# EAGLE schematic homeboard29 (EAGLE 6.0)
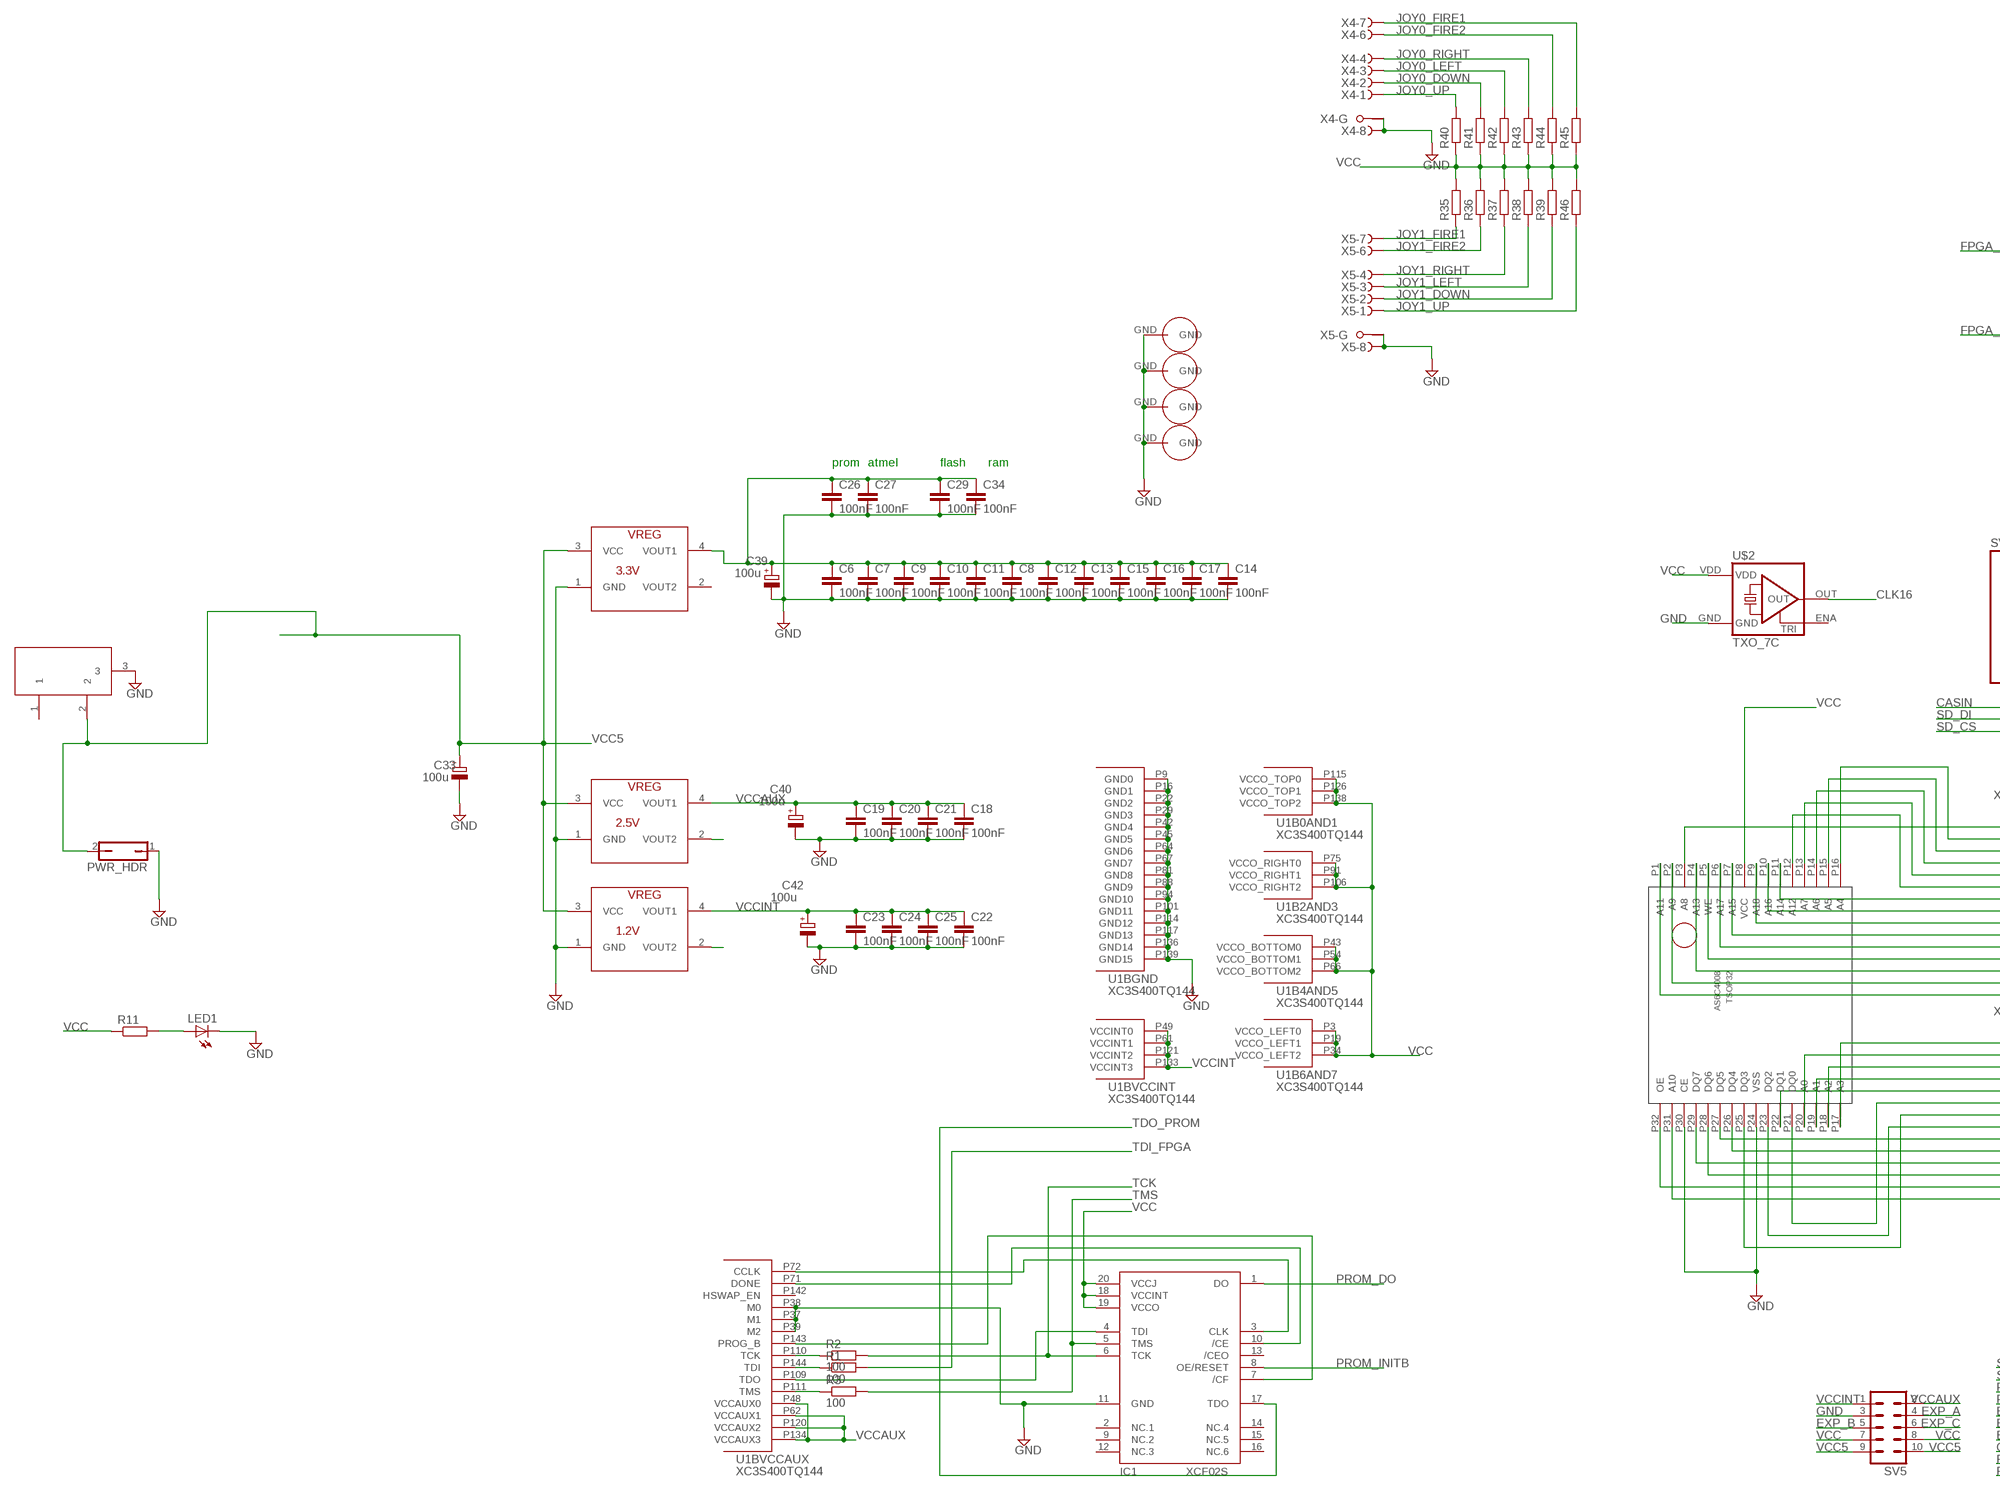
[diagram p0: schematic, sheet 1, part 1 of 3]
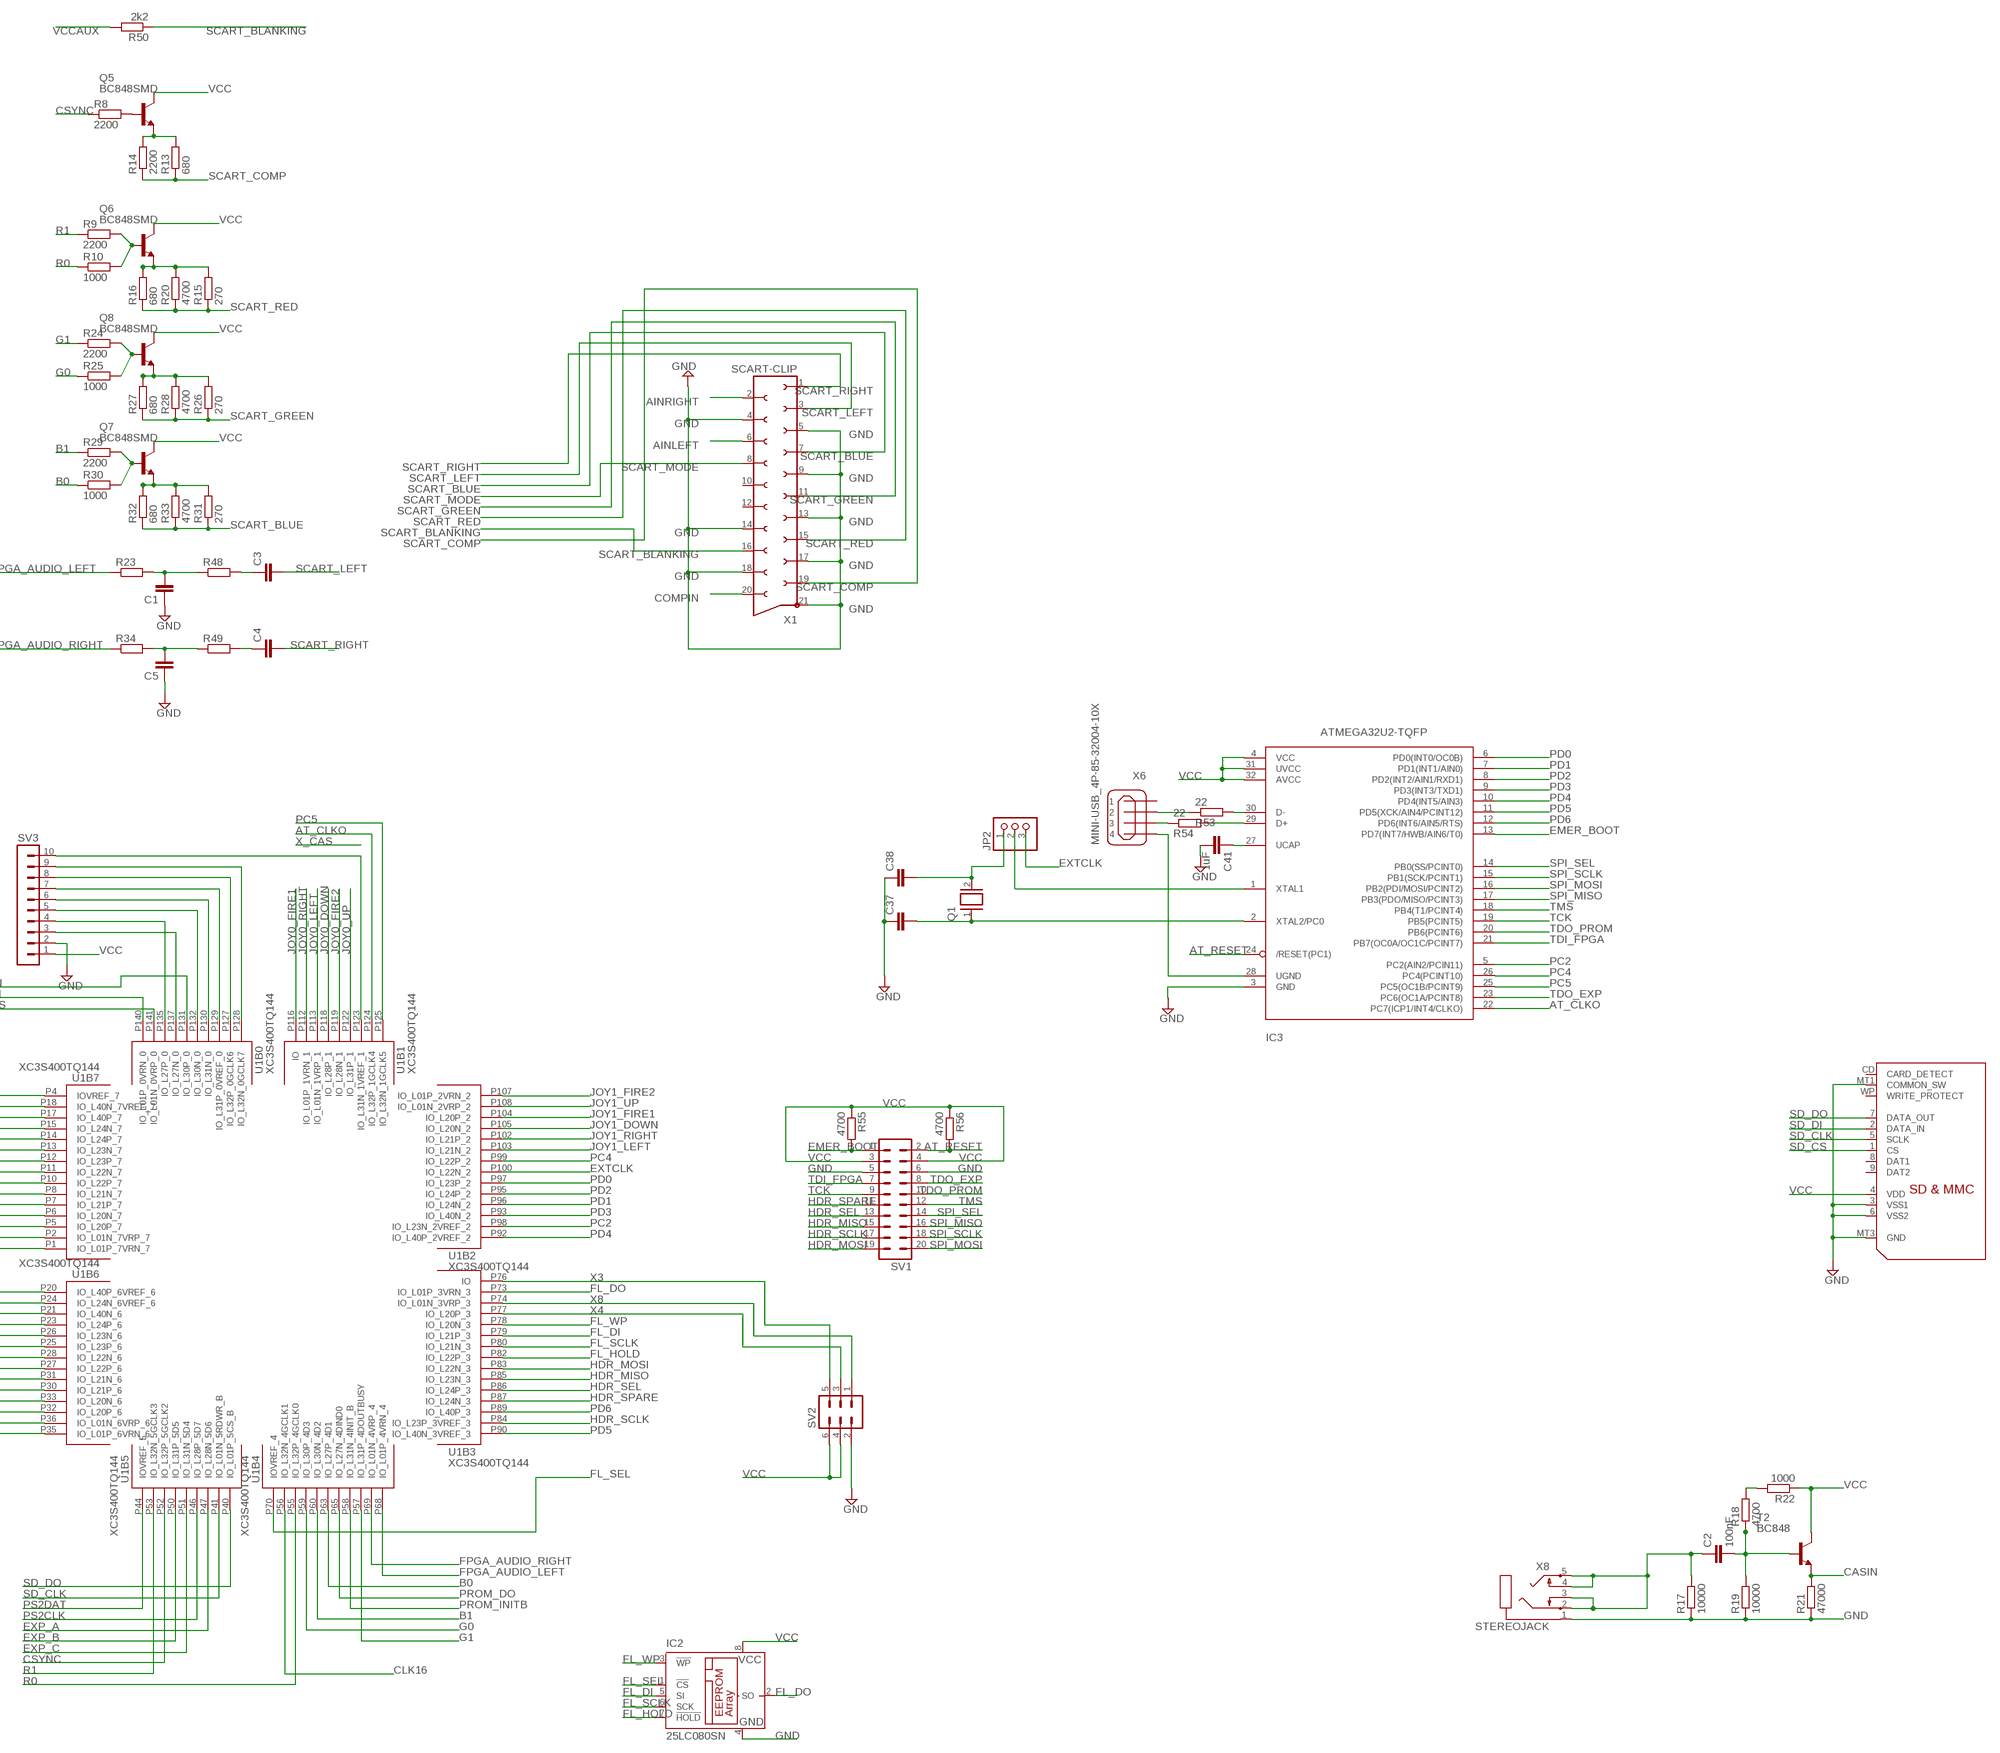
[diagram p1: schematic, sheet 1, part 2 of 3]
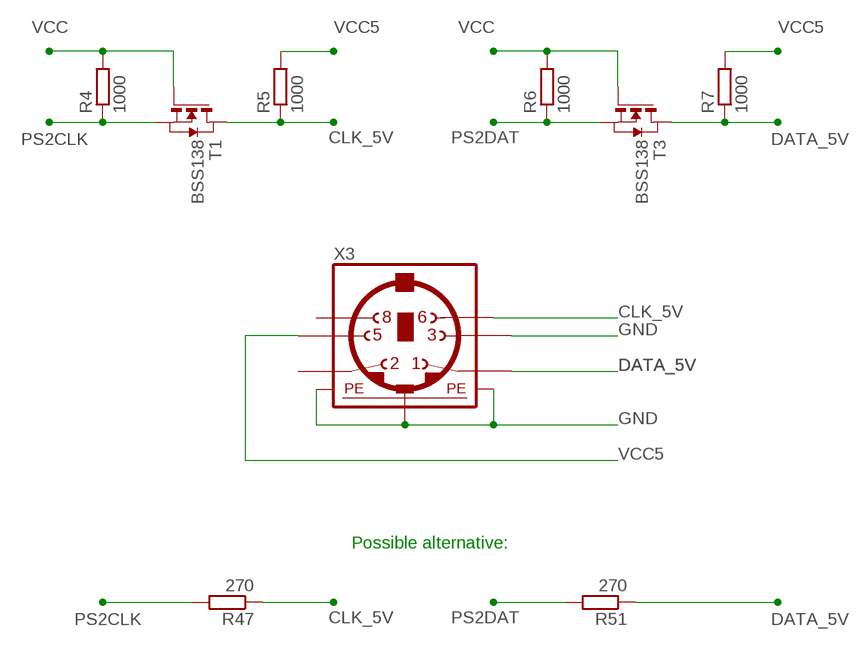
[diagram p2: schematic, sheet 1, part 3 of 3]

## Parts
C1  C-EUC0603  [C0603]
C2  100nF  C-EUC0603  [C0603]
C3  C-EUC0603  [C0603]
C4  C-EUC0603  [C0603]
C5  C-EUC0603  [C0603]
C6  100nF  C-EUC0603  [C0603]
C7  100nF  C-EUC0603  [C0603]
C8  100nF  C-EUC0603  [C0603]
C9  100nF  C-EUC0603  [C0603]
C10  100nF  C-EUC0603  [C0603]
C11  100nF  C-EUC0603  [C0603]
C12  100nF  C-EUC0603  [C0603]
C13  100nF  C-EUC0603  [C0603]
C14  100nF  C-EUC0603  [C0603]
C15  100nF  C-EUC0603  [C0603]
C16  100nF  C-EUC0603  [C0603]
C17  100nF  C-EUC0603  [C0603]
C18  100nF  C-EUC0603  [C0603]
C19  100nF  C-EUC0603  [C0603]
C20  100nF  C-EUC0603  [C0603]
C21  100nF  C-EUC0603  [C0603]
C22  100nF  C-EUC0603  [C0603]
C23  100nF  C-EUC0603  [C0603]
C24  100nF  C-EUC0603  [C0603]
C25  100nF  C-EUC0603  [C0603]
C26  100nF  C-EUC0603  [C0603]
C27  100nF  C-EUC0603  [C0603]
C29  100nF  C-EUC0603  [C0603]
C33  100u  CPOL-EUD  [PANASONIC_D]
C34  100nF  C-EUC0603  [C0603]
C37  C-EUC0805  [C0805]
C38  C-EUC0805  [C0805]
C39  100u  CPOL-EUD  [PANASONIC_D]
C40  100u  CPOL-EUD  [PANASONIC_D]
C41  1uF  C-EUC0805  [C0805]
C42  100u  CPOL-EUD  [PANASONIC_D]
IC1  XCF02S  [VO20]
IC2  25LC080SN  [SO-08]
IC3  ATMEGA32U2-TQFP  [TQFP32-08]
JP2  PINHD-1X3  [1X03]
LED1  LEDCHIPLED_0805  [CHIPLED_0805]
PWR_HDR  JP1Q  [JP1]
Q1  XTAL/S  [QS]
Q5  BC848SMD  [SOT23]
Q6  BC848SMD  [SOT23]
Q7  BC848SMD  [SOT23]
Q8  BC848SMD  [SOT23]
R1  100  R-EU_R0805  [R0805]
R2  100  R-EU_R0805  [R0805]
R3  100  R-EU_R0805  [R0805]
R4  1000  R-EU_R0805  [R0805]
R5  1000  R-EU_R0805  [R0805]
R6  1000  R-EU_R0805  [R0805]
R7  1000  R-EU_R0805  [R0805]
R8  2200  R-EU_R0805  [R0805]
R9  2200  R-EU_R0805  [R0805]
R10  1000  R-EU_R0805  [R0805]
R11  R-EU_M0805  [M0805]
R13  680  R-EU_R0805  [R0805]
R14  2200  R-EU_R0805  [R0805]
R15  270  R-EU_R0805  [R0805]
R16  680  R-EU_R0805  [R0805]
R17  10000  R-EU_R0805  [R0805]
R18  4700  R-EU_R0805  [R0805]
R19  10000  R-EU_R0805  [R0805]
R20  4700  R-EU_R0805  [R0805]
R21  47000  R-EU_R0805  [R0805]
R22  1000  R-EU_R0805  [R0805]
R23  R-EU_M0805  [M0805]
R24  2200  R-EU_R0805  [R0805]
R25  1000  R-EU_R0805  [R0805]
R26  270  R-EU_R0805  [R0805]
R27  680  R-EU_R0805  [R0805]
R28  4700  R-EU_R0805  [R0805]
R29  2200  R-EU_R0805  [R0805]
R30  1000  R-EU_R0805  [R0805]
R31  270  R-EU_R0805  [R0805]
R32  680  R-EU_R0805  [R0805]
R33  4700  R-EU_R0805  [R0805]
R34  R-EU_M0805  [M0805]
R35  R-EU_M0805  [M0805]
R36  R-EU_M0805  [M0805]
R37  R-EU_M0805  [M0805]
R38  R-EU_M0805  [M0805]
R39  R-EU_M0805  [M0805]
R40  R-EU_M0805  [M0805]
R41  R-EU_M0805  [M0805]
R42  R-EU_M0805  [M0805]
R43  R-EU_M0805  [M0805]
R44  R-EU_M0805  [M0805]
R45  R-EU_M0805  [M0805]
R46  R-EU_M0805  [M0805]
R47  270  R-EU_R0805  [R0805]
R48  R-EU_M0805  [M0805]
R49  R-EU_M0805  [M0805]
R50  2k2  R-EU_M0805  [M0805]
R51  270  R-EU_R0805  [R0805]
R53  22  R-EU_R0805  [R0805]
R54  22  R-EU_R0805  [R0805]
R55  4700  R-EU_R0805  [R0805]
R56  4700  R-EU_R0805  [R0805]
REG1.2  1.2V  NX1117  [SOT223]
REG2.5  2.5V  NX1117  [SOT223]
REG3.3  3.3V  NX1117  [SOT223]
SV1  MA10-2  [MA10-2]
SV2  MA03-2  [MA03-2]
SV3  MA10-1  [MA10-1]
SV5  MA05-2  [MA05-2]
T1  BSS138  NMOSSOT23  [SOT-23]
T2  BC848  [SOT23]
T3  BSS138  NMOSSOT23  [SOT-23]
U1  XC3S400TQ144  [TQ144]
U$1  GNDHOLE  [GNDHOLE]
U$2  TXO_7C  [OSC_7C]
U$3  SDMMCNOHOLE  [SDCARD-NOHOLE]
U$6  AS6C4008  [TSOP32]
U$7  GNDHOLE  [GNDHOLE]
U$8  GNDHOLE  [GNDHOLE]
U$9  GNDHOLE  [GNDHOLE]
X1  SCART-CLIP  [SCART-CLIP]
X3  MINI_DIN_6  [M_DIN6]
X4  F09HPS  [F09HP]
X5  F09HPS  [F09HP]
X6  MINI-USB_4P-85-32004-10X  [85-32004-10X]
X7  DC21MMX  [DC-21MM]
X8  STEREOJACK  [20-0137]

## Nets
AINLEFT: X1.6
AINRIGHT: X1.2
AT_CLKO: IC3.22(PC7(ICP1/INT4/CLKO)) U1.P124(B1:IO_L32P_1GCLK4)
AT_RESET: IC3.24(/RESET(PC1)) R56.2 SV1.2
B0: R30.1 U1.P63(B4:IO_L27P_4D1)
B1: R29.1 U1.P60(B4:IO_L30N_4D2)
CASIN: R21.2 T2.2(E) U1.P131(B0:IO_L30P_0)
CLK16: U1.P56(B4:IO_L32N_4GCLK1) U$2.OUT
CLK_5V: R5.1 R47.1 T1.1(D) X3.6
COMPIN: X1.20
CSYNC: R8.1 U1.P52(B5:IO_L32P_5GCLK2)
DATA_5V: R7.1 R51.1 T3.1(D) X3.1
EMER_BOOT: IC3.13(PD7(INT7/HWB/AIN6/T0)) R55.2 SV1.1
EXP_A: SV5.4 U1.P47(B5:IO_L28N_5D6)
EXP_B: SV5.5 U1.P50(B5:IO_L31P_5D5)
EXP_C: SV5.6 U1.P51(B5:IO_L31N_5D4)
EXTCLK: JP2.3 U1.P100(B2:IO_L22N_2)
FL_DI: IC2.5(SI) U1.P79(B3:IO_L21P_3)
FL_DO: IC2.2(SO) U1.P73(B3:IO_L01P_3VRN_3)
FL_HOLD: IC2.7(!HOLD) U1.P82(B3:IO_L22P_3)
FL_SCLK: IC2.6(SCK) U1.P80(B3:IO_L21N_3)
FL_SEL: IC2.1(!CS) U1.P70(B4:IOVREF_4)
FL_WP: IC2.3(!WP) U1.P78(B3:IO_L20N_3)
FPGA_AUDIO_LEFT: R23.1 U1.P68(B4:IO_L01P_4VRN_4)
FPGA_AUDIO_RIGHT: R34.1 U1.P69(B4:IO_L01N_4VRP_4)
G0: R25.1 U1.P59(B4:IO_L30P_4D3)
G1: R24.1 U1.P57(B4:IO_L31P_4DOUTBUSY)
GND: C1.1 C5.1 C6.2 C7.2 C8.2 C9.2 C10.2 C11.2 C12.2 C13.2 C14.2 C15.2 C16.2 C17.2 C18.2 C19.2 C20.2 C21.2 C22.2 C23.2 C24.2 C25.2 C26.2 C27.2 C29.2 C33.- C34.2 C37.1 C38.1 C39.- C40.- C41.2 C42.- IC1.11(GND) IC2.4(GND) IC3.3(GND) LED1.C PWR_HDR.1 R17.1 R19.1 R21.1 REG1.2.1(GND) REG2.5.1(GND) REG3.3.1(GND) SV1.5 SV1.6 SV2.2 SV3.2 SV5.3 U1.P9(BGND:GND0) U1.P16(BGND:GND1) U1.P22(BGND:GND2) U1.P29(BGND:GND3) U1.P37(BVCCAUX:M1) U1.P38(BVCCAUX:M0) U1.P39(BVCCAUX:M2) U1.P42(BGND:GND4) U1.P45(BGND:GND5) U1.P64(BGND:GND6) U1.P67(BGND:GND7) U1.P81(BGND:GND8) U1.P88(BGND:GND9) U1.P94(BGND:GND10) U1.P101(BGND:GND11) U1.P114(BGND:GND12) U1.P117(BGND:GND13) U1.P136(BGND:GND14) U1.P139(BGND:GND15) U$1.GND U$2.GND U$3.3(VSS1) U$3.6(VSS2) U$3.MT1(COMMON_SW) U$3.MT3(GND) U$6.P24(VSS) U$6.P30(CE) U$7.GND U$8.GND U$9.GND X1.4 X1.5 X1.9 X1.13 X1.14 X1.17 X1.18 X1.21 X3.3 X3.SH1(PE1) X3.SH2(PE2) X3.SH3(PE3) X4.8(-8:F) X4.G1(-G:G1) X5.8(-8:F) X5.G1(-G:G1) X7.3 X8.1
HDR_MISO: SV1.15 U1.P85(B3:IO_L23N_3)
HDR_MOSI: SV1.19 U1.P83(B3:IO_L22N_3)
HDR_SCLK: SV1.17 U1.P84(B3:IO_L23P_3VREF_3)
HDR_SEL: SV1.13 U1.P86(B3:IO_L24P_3)
HDR_SPARE: SV1.11 U1.P87(B3:IO_L24N_3)
JOY0_DOWN: R41.2 U1.P118(B1:IO_L28P_1) X4.2(-2:F)
JOY0_FIRE1: R45.2 U1.P116(B1:IO) X4.7(-7:F)
JOY0_FIRE2: R44.2 U1.P119(B1:IO_L28N_1) X4.6(-6:F)
JOY0_LEFT: R42.2 U1.P113(B1:IO_L01N_1VRP_1) X4.3(-3:F)
JOY0_RIGHT: R43.2 U1.P112(B1:IO_L01P_1VRN_1) X4.4(-4:F)
JOY0_UP: R40.2 U1.P122(B1:IO_L31P_1) X4.1(-1:F)
JOY1_DOWN: R39.1 U1.P105(B2:IO_L20N_2) X5.2(-2:F)
JOY1_FIRE1: R35.1 U1.P104(B2:IO_L20P_2) X5.7(-7:F)
JOY1_FIRE2: R36.1 U1.P107(B2:IO_L01P_2VRN_2) X5.6(-6:F)
JOY1_LEFT: R38.1 U1.P103(B2:IO_L21N_2) X5.3(-3:F)
JOY1_RIGHT: R37.1 U1.P102(B2:IO_L21P_2) X5.4(-4:F)
JOY1_UP: R46.1 U1.P108(B2:IO_L01N_2VRP_2) X5.1(-1:F)
N$1: SV3.4 U1.P135(B0:IO_L27P_0)
N$2: SV3.5 U1.P132(B0:IO_L30N_0)
N$3: SV3.3 U1.P137(B0:IO_L27N_0)
N$4: SV3.6 U1.P130(B0:IO_L31N_0)
N$5: SV3.7 U1.P129(B0:IO_L31P_0VREF_0)
N$6: SV3.9 U1.P128(B0:IO_L32N_0GCLK7)
N$7: SV3.8 U1.P127(B0:IO_L32P_0GCLK6)
N$8: IC3.1(XTAL1) JP2.2
N$9: C41.1 IC3.27(UCAP)
N$10: LED1.A R11.2
N$12: C37.2 IC3.2(XTAL2/PC0) Q1.1
N$14: C38.2 JP2.1 Q1.2
N$16: SV3.10 U1.P123(B1:IO_L31N_1VREF_1)
N$35: IC1.3(CLK) U1.P72(BVCCAUX:CCLK)
N$36: R53.1 X6.2
N$38: IC1.10(/CE) U1.P71(BVCCAUX:DONE)
N$39: R2.1 U1.P110(BVCCAUX:TCK)
N$40: IC1.7(/CF) U1.P143(BVCCAUX:PROG_B)
N$42: R1.1 U1.P144(BVCCAUX:TDI)
N$43: R3.1 U1.P111(BVCCAUX:TMS)
N$49: IC3.29(D+) R54.2
N$50: REG2.5.2(VOUT2)
N$51: C1.2 R23.2 R48.1
N$52: C3.1 R48.2
N$53: Q6.1(B) R9.2 R10.2
N$54: Q6.2(E) R15.2 R16.2 R20.2
N$55: Q8.1(B) R24.2 R25.2
N$56: Q8.2(E) R26.2 R27.2 R28.2
N$57: Q7.1(B) R29.2 R30.2
N$58: Q7.2(E) R31.2 R32.2 R33.2
N$59: Q5.2(E) R13.2 R14.2
N$60: C2.2 R18.1 R19.2 T2.1(B)
N$61: C2.1 R17.2 X8.2 X8.3 X8.4 X8.5
N$62: R18.2 R22.2
N$63: Q5.1(B) R8.2
N$64: C4.1 R49.2
N$65: C5.2 R34.2 R49.1
N$66: R54.1 X6.3
N$67: U1.P1(B7:IO_L01P_7VRN_7) U$6.P1(A11)
N$68: IC3.30(D-) R53.2
N$69: IC3.28(UGND) X6.4
N$70: REG1.2.2(VOUT2)
N$71: U1.P2(B7:IO_L01N_7VRP_7) U$6.P2(A9)
N$72: U1.P4(B7:IOVREF_7) U$6.P3(A8)
N$73: U1.P5(B7:IO_L20P_7) U$6.P4(A13)
N$74: U1.P6(B7:IO_L20N_7) U$6.P5(WE)
N$75: U1.P7(B7:IO_L21P_7) U$6.P6(A17)
N$76: U1.P8(B7:IO_L21N_7) U$6.P7(A15)
N$77: U1.P10(B7:IO_L22P_7) U$6.P9(A18)
N$78: U1.P11(B7:IO_L22N_7) U$6.P10(A16)
N$79: U1.P12(B7:IO_L23P_7) U$6.P11(A14)
N$80: U1.P13(B7:IO_L23N_7) U$6.P12(A12)
N$81: U1.P14(B7:IO_L24P_7) U$6.P13(A7)
N$82: U1.P15(B7:IO_L24N_7) U$6.P14(A6)
N$83: U1.P17(B7:IO_L40P_7) U$6.P15(A5)
N$84: U1.P18(B7:IO_L40N_7VREF_7) U$6.P16(A4)
N$85: U1.P20(B6:IO_L40P_6VREF_6) U$6.P17(A3)
N$86: U1.P21(B6:IO_L40N_6) U$6.P18(A2)
N$87: U1.P23(B6:IO_L24P_6) U$6.P19(A1)
N$88: U1.P24(B6:IO_L24N_6VREF_6) U$6.P20(A0)
N$89: U1.P25(B6:IO_L23P_6) U$6.P21(DQ0)
N$90: U1.P26(B6:IO_L23N_6) U$6.P22(DQ1)
N$91: U1.P27(B6:IO_L22P_6) U$6.P23(DQ2)
N$92: U1.P28(B6:IO_L22N_6) U$6.P25(DQ3)
N$93: U1.P30(B6:IO_L21P_6) U$6.P26(DQ4)
N$94: U1.P31(B6:IO_L21N_6) U$6.P27(DQ5)
N$95: U1.P32(B6:IO_L20P_6) U$6.P28(DQ6)
N$96: U1.P33(B6:IO_L20N_6) U$6.P29(DQ7)
N$97: U1.P35(B6:IO_L01P_6VRN_6) U$6.P31(A10)
N$98: U1.P36(B6:IO_L01N_6VRP_6) U$6.P32(OE)
PC2: IC3.5(PC2(AIN2/PCIN11)) U1.P98(B2:IO_L23N_2VREF_2)
PC4: IC3.26(PC4(PCINT10)) U1.P99(B2:IO_L22P_2)
PC5: IC3.25(PC5(OC1B/PCINT9)) U1.P125(B1:IO_L32N_1GCLK5)
PD0: IC3.6(PD0(INT0/OC0B)) U1.P97(B2:IO_L23P_2)
PD1: IC3.7(PD1(INT1/AIN0)) U1.P96(B2:IO_L24N_2)
PD2: IC3.8(PD2(INT2/AIN1/RXD1)) U1.P95(B2:IO_L24P_2)
PD3: IC3.9(PD3(INT3/TXD1)) U1.P93(B2:IO_L40N_2)
PD4: IC3.10(PD4(INT5/AIN3)) U1.P92(B2:IO_L40P_2VREF_2)
PD5: IC3.11(PD5(XCK/AIN4/PCINT12)) U1.P90(B3:IO_L40N_3VREF_3)
PD6: IC3.12(PD6(INT6/AIN5/RTS)) U1.P89(B3:IO_L40P_3)
PROM_DO: IC1.1(DO) U1.P65(B4:IO_L27N_4DIND0)
PROM_INITB: IC1.8(OE/RESET) U1.P58(B4:IO_L31N_4INIT_B)
PS2CLK: R4.1 R47.2 T1.2(S) U1.P46(B5:IO_L28P_5D7)
PS2DAT: R6.1 R51.2 T3.2(S) U1.P44(B5:IOVREF_5)
R0: R10.1 U1.P55(B4:IO_L32P_4GCLK0)
R1: R9.1 U1.P53(B5:IO_L32N_5GCLK3)
SCART_BLANKING: R50.1 X1.16
SCART_BLUE: R31.1 R32.1 R33.1 X1.7
SCART_COMP: R13.1 R14.1 X1.19
SCART_GREEN: R26.1 R27.1 R28.1 X1.11
SCART_LEFT: C3.2 X1.3
SCART_MODE: X1.8
SCART_RED: R15.1 R16.1 R20.1 X1.15
SCART_RIGHT: C4.2 X1.1
SD_CLK: U1.P41(B5:IO_L01N_5RDWR_B) U$3.5(SCLK)
SD_CS: U1.P141(B0:IO_L01N_0VRP_0) U$3.1(CS)
SD_DI: U1.P140(B0:IO_L01P_0VRN_0) U$3.2(DATA_IN)
SD_DO: U1.P40(B5:IO_L01P_5CS_B) U$3.7(DATA_OUT)
SPI_MISO: IC3.17(PB3(PDO/MISO/PCINT3)) SV1.16
SPI_MOSI: IC3.16(PB2(PDI/MOSI/PCINT2)) SV1.20
SPI_SCLK: IC3.15(PB1(SCK/PCINT1)) SV1.18
SPI_SEL: IC3.14(PB0(SS/PCINT0)) SV1.14
TCK: IC1.6(TCK) IC3.19(PB5(PCINT5)) R2.2 SV1.9
TDI_FPGA: IC3.21(PB7(OC0A/OC1C/PCINT7)) R1.2 SV1.7
TDO_EXP: IC3.23(PC6(OC1A/PCINT8)) SV1.8
TDO_FPGA: IC1.4(TDI) U1.P109(BVCCAUX:TDO)
TDO_PROM: IC1.17(TDO) IC3.20(PB6(PCINT6)) SV1.10
TMS: IC1.5(TMS) IC3.18(PB4(T1/PCINT4)) R3.2 SV1.12
VCC: C6.1 C7.1 C8.1 C9.1 C10.1 C11.1 C12.1 C13.1 C14.1 C15.1 C16.1 C17.1 C26.1 C27.1 C29.1 C34.1 C39.+ IC1.18(VCCINT) IC1.19(VCCO) IC1.20(VCCJ) IC2.8(VCC) IC3.4(VCC) IC3.31(UVCC) IC3.32(AVCC) Q5.3(C) Q6.3(C) Q7.3(C) Q8.3(C) R4.2 R6.2 R11.1 R22.1 R35.2 R36.2 R37.2 R38.2 R39.2 R40.1 R41.1 R42.1 R43.1 R44.1 R45.1 R46.2 R55.1 R56.1 REG3.3.4(VOUT1) SV1.3 SV1.4 SV2.4 SV2.6 SV3.1 SV5.7 SV5.8 T1.3(G) T2.3(C) T3.3(G) U1.P3(B6AND7:VCCO_LEFT0) U1.P19(B6AND7:VCCO_LEFT1) U1.P34(B6AND7:VCCO_LEFT2) U1.P43(B4AND5:VCCO_BOTTOM0) U1.P54(B4AND5:VCCO_BOTTOM1) U1.P66(B4AND5:VCCO_BOTTOM2) U1.P75(B2AND3:VCCO_RIGHT0) U1.P91(B2AND3:VCCO_RIGHT1) U1.P106(B2AND3:VCCO_RIGHT2) U1.P115(B0AND1:VCCO_TOP0) U1.P126(B0AND1:VCCO_TOP1) U1.P138(B0AND1:VCCO_TOP2) U$2.VDD U$3.4(VDD) U$6.P8(VCC)
VCC5: C33.+ PWR_HDR.2 R5.2 R7.2 REG1.2.3(VCC) REG2.5.3(VCC) REG3.3.3(VCC) SV5.9 SV5.10 X3.5 X7.2
VCCAUX: C18.1 C19.1 C20.1 C21.1 C40.+ R50.2 REG2.5.4(VOUT1) SV5.2 U1.P48(BVCCAUX:VCCAUX0) U1.P62(BVCCAUX:VCCAUX1) U1.P120(BVCCAUX:VCCAUX2) U1.P134(BVCCAUX:VCCAUX3)
VCCINT: C22.1 C23.1 C24.1 C25.1 C42.+ REG1.2.4(VOUT1) SV5.1 U1.P49(BVCCINT:VCCINT0) U1.P61(BVCCINT:VCCINT1) U1.P121(BVCCINT:VCCINT2) U1.P133(BVCCINT:VCCINT3)
X3: SV2.5 U1.P76(B3:IO)
X4: SV2.3 U1.P77(B3:IO_L20P_3)
X8: SV2.1 U1.P74(B3:IO_L01N_3VRP_3)
Unconnected: IC1.2(NC.1) IC1.9(NC.2) IC1.12(NC.3) IC1.13(/CEO) IC1.14(NC.4) IC1.15(NC.5) IC1.16(NC.6) REG3.3.2(VOUT2) U1.P142(BVCCAUX:HSWAP_EN) U$2.ENA(TRI) U$3.8(DAT1) U$3.9(DAT2) U$3.CD(CARD_DETECT) U$3.WP(WRITE_PROTECT) X1.10 X1.12 X3.2 X3.8 X4.5(-5:F) X4.9(-9:F) X4.G2(-G:G2) X5.5(-5:F) X5.9(-9:F) X5.G2(-G:G2) X6.1

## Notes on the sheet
- prom | atmel | flash | ram
- Possible alternative:

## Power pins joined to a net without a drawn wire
1: X7.1

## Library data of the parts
C1-C5 = resistor:C-EU: CAPACITOR, European symbol
C6-C27 C29 C34 C37 C38 C41 = rcl:C-EU: CAPACITOR, European symbol
C33 C39 C40 C42 = rcl:CPOL-EU: POLARIZED CAPACITOR, European symbol
IC1 = smd-special:XCF02S
IC2 = microchip:25*: Serial EEPROM 4K/ 8K , SPI bus; MF: MICROCHIP; MPN: 25LC080/SN; OC_FARNELL: 1137302; OC_NEWARK: 96K4092
IC3 = adafruit:ATMEGA32U2: ATmega32u2 Pin compatible with the atmega8u2, atmega16u2 and atmega32u2 8, 16 or 32 K flash, 1K RAM, 512b EEPROM 8 bit and 16 bit timer (5 PWM total) UART, SPI (no I2C!) USB with 4 endpoints, LUFA compatible 22 I/O lines, analog comparator (no ADC!) Comes with DFU bootloader burned in!
JP2 = adafruit:PINHD-1X3: PIN HEADER
LED1 = adafruit:LED: LED
PWR_HDR = jumper:JP1Q: JUMPER
Q1 = special:XTAL/S: CRYSTAL
Q5-Q8 = bc548:BC848*: NPN Transistor
R1-R10 R13-R22 R24-R33 R47 R51 R53-R56 = rcl:R-EU_: RESISTOR, European symbol
R11 R23 R34-R46 R48-R50 = resistor:R-EU_: RESISTOR, European symbol
REG1.2 REG2.5 REG3.3 = cpcfpga:NX1117
SV1 = con-lstb:MA10-2: PIN HEADER; OC_FARNELL: unknown; OC_NEWARK: unknown
SV2 = con-lstb:MA03-2: PIN HEADER; OC_FARNELL: unknown; OC_NEWARK: unknown
SV3 = con-lstb:MA10-1: PIN HEADER; OC_FARNELL: unknown; OC_NEWARK: unknown
SV5 = con-lstb:MA05-2: PIN HEADER; OC_FARNELL: unknown; OC_NEWARK: unknown
T1 T3 = zetex:NMOSSOT23: MOS FET; OC_FARNELL: unknown; OC_NEWARK: unknown
T2 = transistor:BC848: NPN TRANSISTOR
U1 = xilinx_spartan3_virtex4_and_5:XC3S400TQ144: Xilinx FPGA
U$1 U$7-U$9 = cpcfpga:GNDHOLE
U$2 = cpcfpga:TXO_7C: TXC crystal oscillator http://www.txccrystal.com/images/pdf/7c.pdf
U$3 = cpcfpga:SDMMC: SD MMC Card holder 4UCON part #06132 - easy to solder
U$6 = cpcfpga:AS6C4008
X1 = cpcfpga:SCART-CLIP: TV SCART CONNECTOR; OC_FARNELL: unknown; OC_NEWARK: unknown
X3 = mini_din:MINI_DIN_6
X4 X5 = con-subd:F09HPS: SUB-D; OC_FARNELL: unknown; OC_NEWARK: unknown
X6 = con-cypressindustries:MINI-USB_4P-: MINI USB 4 Pol. Source: www.cypressindustries.com; OC_FARNELL: unknown; OC_NEWARK: unknown
X7 = powersupply:DC21MM
X8 = cpcfpga:STEREOJACK: MIC/HEADPHONE JACK Stereo jack with two switches. Kycon STX3100, CUI SJ1-3555NG and/or 4UCon 05544 modified from adafruit library

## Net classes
1 power: width 0.6 mm, drill 1.1 mm, clearance 0.4 mm
2 gnd: width 0.305 mm, drill 0.508 mm, clearance 0.152 mm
